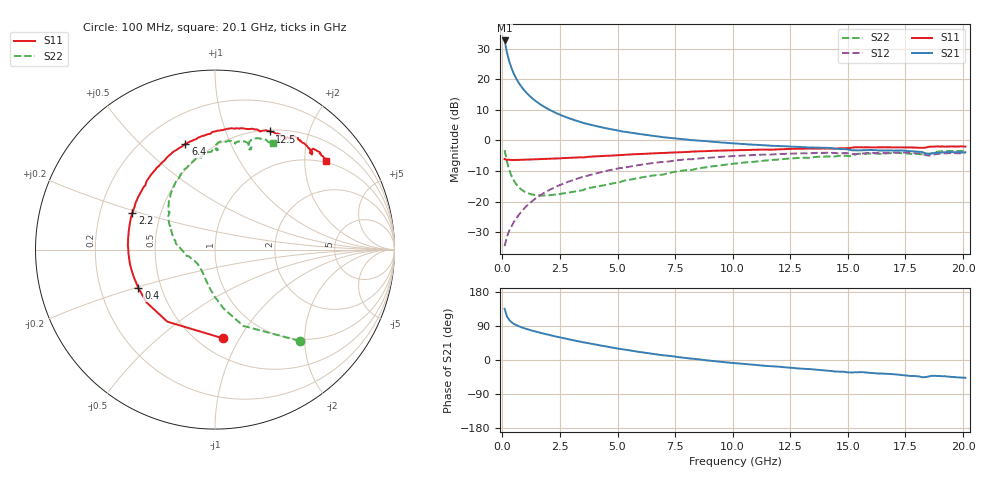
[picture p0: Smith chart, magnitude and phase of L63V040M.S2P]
!  Infineon Technologies AG
! BFR380L3 , PF131585-7, No.6, Th 09.10.01, soldered on pcb-board, measured with PP GSG850
!  Vce=3.0 V,  Ic=40.0 mA
! Common Emitter S-Parameters:  15. November 2001
#  GHz  S  MA  R  50
! f  S11  S21  S12  S22
! GHz  Mag  Ang  Mag  Ang  Mag  Ang  Mag  Ang
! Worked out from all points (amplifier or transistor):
!   201 points, 100 MHz to 20.1 GHz, reference 50 ohm
!   highest |S21| = 32.7 dB at 100 MHz (marker M1)
!   |S21| within 3 dB of that: start of sweep to 177.5 MHz
!   unconditionally stable (mu >= 1): 1.091 GHz to 4.246 GHz
!   at 3.4 GHz: K = 1.01, MAG = 8.3 dB, |S12| = -12.1 dB
!   at 10.1 GHz: K = 0.96, MSG = 2.1 dB, |S12| = -5.1 dB
!   at 20.1 GHz: K = 0.99, MSG = 0.1 dB, |S12| = -4.1 dB
!   S11 on the Smith chart (normalised r, x): 100 MHz: 0.65, -0.86; 400 MHz: 0.37, -0.21; 2.2 GHz: 0.34, +0.19; 6.4 GHz: 0.37, +0.69; 12.5 GHz: 0.52, +1.44; 20.1 GHz: 0.96, +2.54
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0.1  0.4967 -84.8  42.95 135.2  0.01868 63.5  0.6933 -47.2
0.2  0.4815 -123.5  27.51 115.2  0.02664 57.2  0.4533 -69.6
0.3  0.4818 -142.4  19.59 105.7  0.03349 59.0  0.331 -81.8
0.4  0.4774 -153.3  15.11 99.7  0.03954 61.5  0.2626 -90.3
0.5  0.4774 -160.9  12.26 95.4  0.04627 63.5  0.2211 -97.0
0.6  0.4789 -166.5  10.3 92.2  0.05276 65.0  0.1932 -102.5
0.7  0.4809 -170.8  8.887 89.5  0.0595 66.1  0.1741 -107.5
0.8  0.4813 -174.4  7.803 87.0  0.06667 67.1  0.1602 -111.8
1  0.4833 179.5  6.29 82.8  0.08086 67.9  0.143 -119.4
1.2  0.4864 174.6  5.27 79.2  0.095 68.1  0.1335 -125.9
1.5  0.4915 168.2  4.251 74.1  0.1163 67.6  0.1268 -133.9
1.8  0.4962 162.8  3.57 69.5  0.1377 66.5  0.1255 -140.7
2.2  0.5038 156.1  2.957 63.8  0.1657 64.5  0.1291 -148.4
3.5  0.528 137.3  1.94 46.9  0.2539 56.3  0.1536 -166.6
4.9  0.5689 120.8  1.476 31.4  0.34 46.6  0.2008 174.8
6.4  0.6111 105.7  1.206 17.2  0.42 36.0  0.2617 157.8
6.8  0.6195 101.9  1.153 14.0  0.4388 32.9  0.2739 153.2
10.1  0.6921 77.8  0.8919 -8.3  0.5555 11.3  0.4177 123.9
12.5  0.7254 65.2  0.792 -20.5  0.6097 -3.3  0.5049 104.4
13.5  0.7355 60.5  0.7654 -24.9  0.6197 -9.2  0.5295 97.8
16.8  0.771 48.2  0.6831 -36.4  0.6263 -25.0  0.618 77.4
20.1  0.7917 38.6  0.6406 -47.0  0.6203 -38.6  0.6751 61.5
